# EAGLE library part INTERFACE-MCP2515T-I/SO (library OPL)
Stand-Alone CAN Controller with SPI Interface
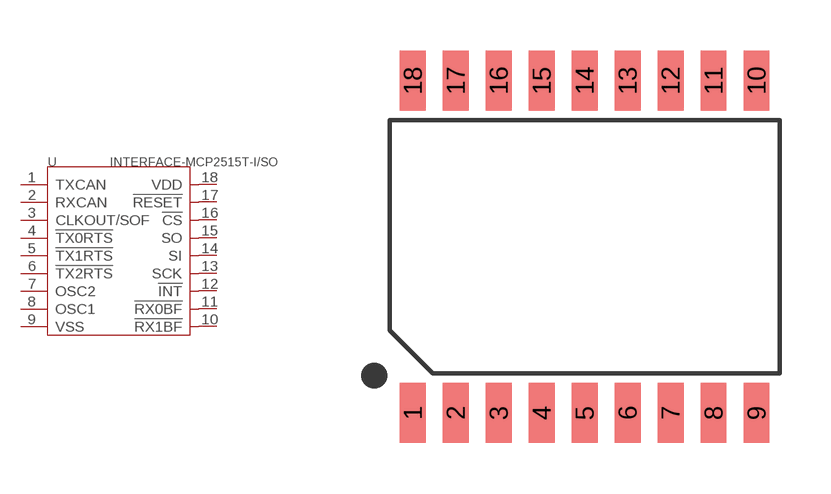
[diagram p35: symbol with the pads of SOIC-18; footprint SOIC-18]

Designator prefix U

## INTERFACE-MCP2515T-I/SO-310070025  [SOIC-18]
1  TXCAN  out
2  RXCAN  in
3  CLKOUT/SOF  out
4  !TX0RTS  in
5  !TX1RTS  in
6  !TX2RTS  in
7  OSC2  out
8  OSC1  in
9  VSS  sup
10  !RX1BF  out
11  !RX0BF  out
12  !INT  out
13  SCK  in
14  SI  in
15  SO  out
16  !CS  in
17  !RESET  in
18  VDD  sup

## Footprint SOIC-18 (pad centres in mm)
smd 0.762 x 1.778: 1 -5.08,-4.915; 2 -3.81,-4.915; 3 -2.54,-4.915; 4 -1.27,-4.915; 5 0,-4.915; 6 1.27,-4.915; 7 2.54,-4.915; 8 3.81,-4.915; 9 5.08,-4.915; 10 5.08,4.915; 11 3.81,4.915; 12 2.54,4.915; 13 1.27,4.915; 14 0,4.915; 15 -1.27,4.915; 16 -2.54,4.915; 17 -3.81,4.915; 18 -5.08,4.915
